// ------------------------------------------------------------------
// File           : C:\Programmi\Siemens\NCVar Selector\ASSI2.awl
//
// Source File    : C:\Programmi\Siemens\NCVar Selector\ASSI2.var
// Generation Date: 16/10/2015  Time: 18.39.23
// ------------------------------------------------------------------

DATA_BLOCK DB  123
VERSION : 0.0


STRUCT

 C1_SGA_actToolBasePos1_2:
   STRUCT
   SYNTAX_ID : BYTE  := B#16#82;
   bereich_u_einheit : BYTE := B#16#41;
   spalte : WORD := W#16#2;
   zeile : WORD := W#16#1;
   bausteintyp : BYTE := B#16#73;
   ZEILENANZAHL : BYTE := B#16#1;
   typ : BYTE := B#16#F;
   laenge : BYTE := B#16#8;
   END_STRUCT ;

 C1_SGA_actToolBasePos2_2:
   STRUCT
   SYNTAX_ID : BYTE  := B#16#82;
   bereich_u_einheit : BYTE := B#16#41;
   spalte : WORD := W#16#2;
   zeile : WORD := W#16#2;
   bausteintyp : BYTE := B#16#73;
   ZEILENANZAHL : BYTE := B#16#1;
   typ : BYTE := B#16#F;
   laenge : BYTE := B#16#8;
   END_STRUCT ;

 C1_SGA_actToolBasePos3_2:
   STRUCT
   SYNTAX_ID : BYTE  := B#16#82;
   bereich_u_einheit : BYTE := B#16#41;
   spalte : WORD := W#16#2;
   zeile : WORD := W#16#3;
   bausteintyp : BYTE := B#16#73;
   ZEILENANZAHL : BYTE := B#16#1;
   typ : BYTE := B#16#F;
   laenge : BYTE := B#16#8;
   END_STRUCT ;

 C2_SGA_actToolBasePos1_2:
   STRUCT
   SYNTAX_ID : BYTE  := B#16#82;
   bereich_u_einheit : BYTE := B#16#42;
   spalte : WORD := W#16#2;
   zeile : WORD := W#16#1;
   bausteintyp : BYTE := B#16#73;
   ZEILENANZAHL : BYTE := B#16#1;
   typ : BYTE := B#16#F;
   laenge : BYTE := B#16#8;
   END_STRUCT ;

 C2_SGA_actToolBasePos2_2:
   STRUCT
   SYNTAX_ID : BYTE  := B#16#82;
   bereich_u_einheit : BYTE := B#16#42;
   spalte : WORD := W#16#2;
   zeile : WORD := W#16#2;
   bausteintyp : BYTE := B#16#73;
   ZEILENANZAHL : BYTE := B#16#1;
   typ : BYTE := B#16#F;
   laenge : BYTE := B#16#8;
   END_STRUCT ;

 C2_SGA_actToolBasePos3_2:
   STRUCT
   SYNTAX_ID : BYTE  := B#16#82;
   bereich_u_einheit : BYTE := B#16#42;
   spalte : WORD := W#16#2;
   zeile : WORD := W#16#3;
   bausteintyp : BYTE := B#16#73;
   ZEILENANZAHL : BYTE := B#16#1;
   typ : BYTE := B#16#F;
   laenge : BYTE := B#16#8;
   END_STRUCT ;

 END_STRUCT ;

BEGIN
END_DATA_BLOCK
